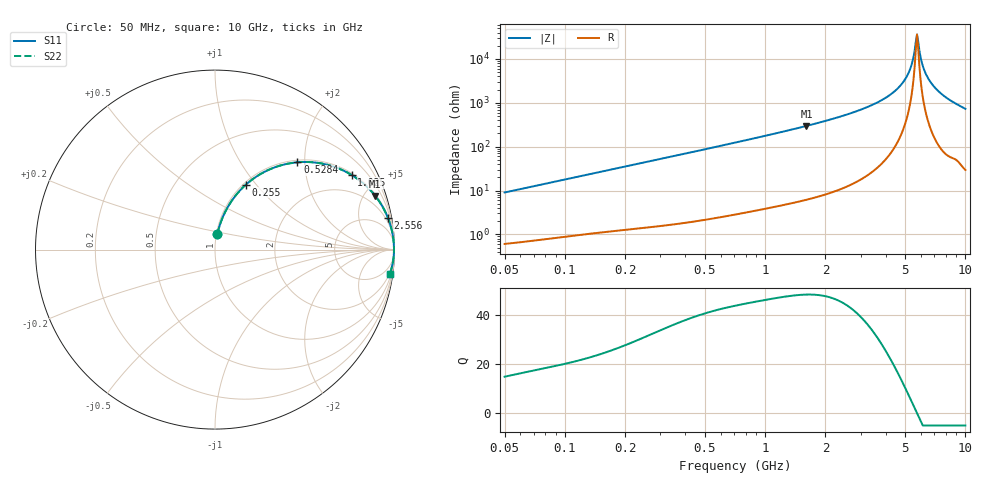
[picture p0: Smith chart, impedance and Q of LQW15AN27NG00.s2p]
!Murata Part Number: LQW15AN27NG00
!These Parameters are Measured in Series Mode Connection
!  o--[Z]--o
!Port1  Port2
!  o-------o
!Freq. Start=50[MHz] Stop=10[GHz], 401[Steps]
# Hz S RI R 50
!Freq.(Hz)	S 11(Real)	S 11(Imag)	S 21(Real)	S 21(Imag)	S 12(Real)	S 12(Imag)	S 22(Real)	S 22(Imag)
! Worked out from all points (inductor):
!   401 points, 50 MHz to 10 GHz, reference 50 ohm
!   read as one part in series: L = 28.5 nH near 51.34 MHz
!   highest Q = 48.3 at 1.607 GHz (marker M1), where L = 29.4 nH
!   self-resonance near 5.733 GHz
!   S11 on the Smith chart (normalised r, x): 50 MHz: 1.01, +0.18; 255 MHz: 1.03, +0.89; 528.4 MHz: 1.04, +1.84; 1.025 GHz: 1.08, +3.62; 2.556 GHz: 1, +11; 10 GHz: 2, -15
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5e7  0.0139 0.0881  0.9861 -0.0881  0.9861 -0.0881  0.0139 0.0881
1.214486e8  0.0524 0.2012  0.9476 -0.2012  0.9476 -0.2012  0.0524 0.2012
2.54998e8  0.1729 0.3625  0.8271 -0.3625  0.8271 -0.3625  0.1729 0.3625
2.949953e8  0.2158 0.3967  0.7842 -0.3967  0.7842 -0.3967  0.2158 0.3967
5.283581e8  0.4592 0.4863  0.5408 -0.4863  0.5408 -0.4863  0.4592 0.4863
7.071068e8  0.6017 0.4783  0.3983 -0.4783  0.3983 -0.4783  0.6017 0.4783
1.024606e9  0.7617 0.4154  0.2383 -0.4154  0.2383 -0.4154  0.7617 0.4154
1.607477e9  0.8932 0.2987  0.1068 -0.2987  0.1068 -0.2987  0.8932 0.2987
1.717543e9  0.9067 0.2807  0.0933 -0.2807  0.0933 -0.2807  0.9067 0.2807
2.555552e9  0.963 0.1778  0.037 -0.1778  0.037 -0.1778  0.963 0.1778
4.171863e9  0.9926 0.0668  0.00745 -0.0668  0.00745 -0.0668  0.9926 0.0668
4.700058e9  0.9954 0.0417  0.00457 -0.0417  0.00457 -0.0417  0.9954 0.0417
5.088839e9  0.9966 0.0251  0.0034 -0.0251  0.0034 -0.0251  0.9966 0.0251
5.365732e9  0.997 0.014  0.00295 -0.014  0.00295 -0.014  0.997 0.014
5.583245e9  0.9972 0.00564  0.00278 -0.00564  0.00278 -0.00564  0.9972 0.00564
5.733131e9  0.9972 5.6e-05  0.00276 -5.6e-05  0.00276 -5.6e-05  0.9972 5.6e-05
5.88704e9  0.9972 -0.00555  0.0028 0.00555  0.0028 0.00555  0.9972 -0.00555
6.045081e9  0.9971 -0.0112  0.00291 0.0112  0.00291 0.0112  0.9971 -0.0112
6.207365e9  0.9969 -0.0169  0.00309 0.0169  0.00309 0.0169  0.9969 -0.0169
6.810442e9  0.9957 -0.0371  0.00432 0.0371  0.00432 0.0371  0.9957 -0.0371
7.983737e9  0.9907 -0.0738  0.00926 0.0738  0.00926 0.0738  0.9907 -0.0738
1e10  0.9762 -0.1334  0.0238 0.1334  0.0238 0.1334  0.9762 -0.1334
